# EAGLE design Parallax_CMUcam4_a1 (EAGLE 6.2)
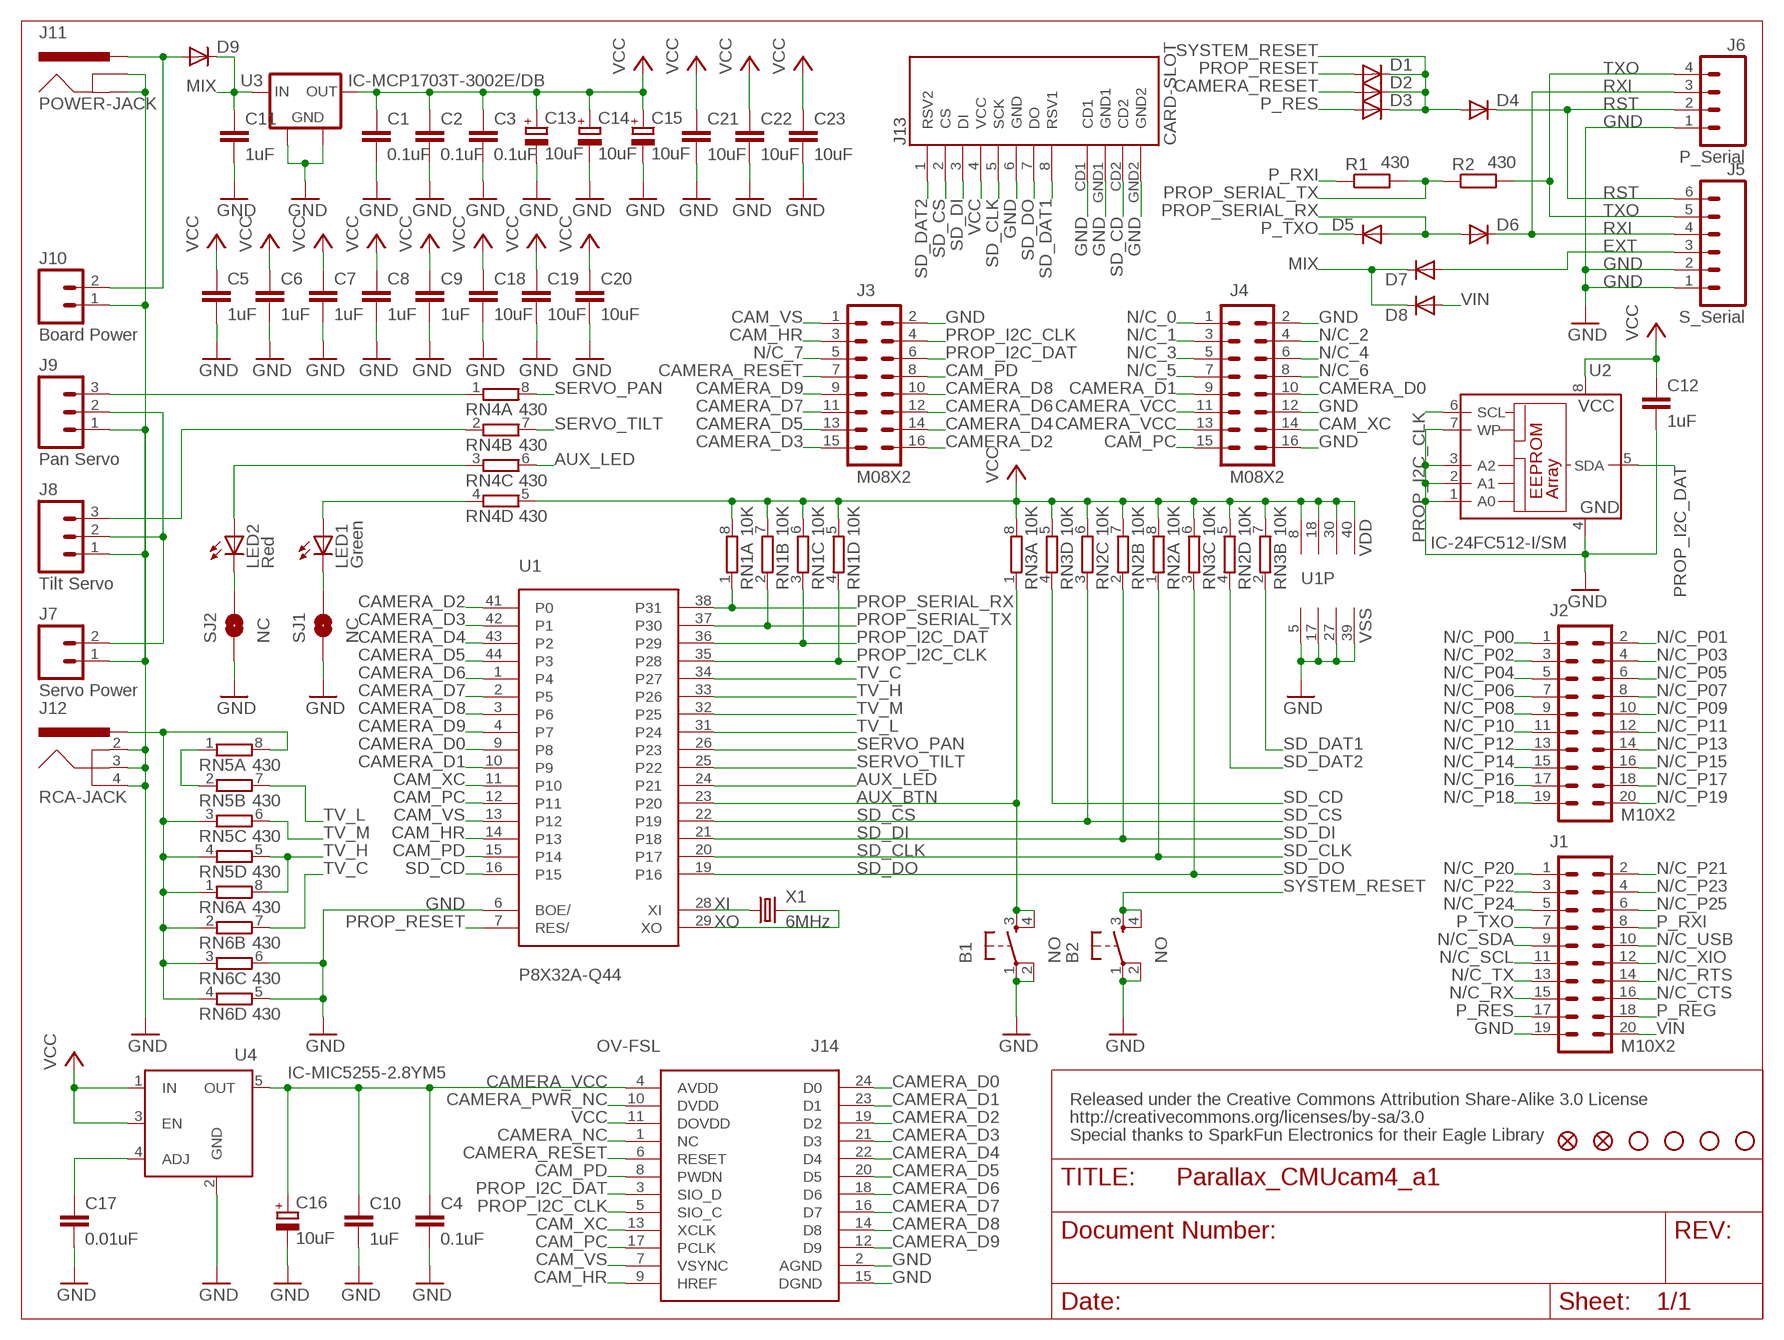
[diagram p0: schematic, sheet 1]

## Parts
B1  NO  PUSH-BUTTON  [PUSH-BUTTON]
B2  NO  PUSH-BUTTON  [PUSH-BUTTON]
C1  0.1uF  C-EUC0603K  [C0603K]
C2  0.1uF  C-EUC0603K  [C0603K]
C3  0.1uF  C-EUC0603K  [C0603K]
C4  0.1uF  C-EUC0603K  [C0603K]
C5  1uF  C-EUC0603K  [C0603K]
C6  1uF  C-EUC0603K  [C0603K]
C7  1uF  C-EUC0603K  [C0603K]
C8  1uF  C-EUC0603K  [C0603K]
C9  1uF  C-EUC0603K  [C0603K]
C10  1uF  C-EUC0603K  [C0603K]
C11  1uF  C-EUC0603K  [C0603K]
C12  1uF  C-EUC0603K  [C0603K]
C13  10uF  CPOL-EUA/3216-18R  [A/3216-18R]
C14  10uF  CPOL-EUA/3216-18R  [A/3216-18R]
C15  10uF  CPOL-EUA/3216-18R  [A/3216-18R]
C16  10uF  CPOL-EUA/3216-18R  [A/3216-18R]
C17  0.01uF  C-EUC0603K  [C0603K]
C18  10uF  C-EUC0603K  [C0603K]
C19  10uF  C-EUC0603K  [C0603K]
C20  10uF  C-EUC0603K  [C0603K]
C21  10uF  C-EUC0603K  [C0603K]
C22  10uF  C-EUC0603K  [C0603K]
C23  10uF  C-EUC0603K  [C0603K]
D1  DIODE-SOD523  [SOD523]
D2  DIODE-SOD523  [SOD523]
D3  DIODE-SOD523  [SOD523]
D4  DIODE-SOD523  [SOD523]
D5  DIODE-SOD523  [SOD523]
D6  DIODE-SOD523  [SOD523]
D7  DIODE-SOD323-R  [SOD323]
D8  DIODE-SOD323-R  [SOD323]
D9  DIODE-SOD323-R  [SOD323]
FID1  FIDUCIAL1X2  [FIDUCIAL-1X2]
FID2  FIDUCIAL1X2  [FIDUCIAL-1X2]
J1  M10X2  [2X10]
J2  M10X2  [2X10]
J3  M08X2  [2X8]
J4  M08X2  [2X8]
J5  S_Serial  M06SIP  [1X06]
J6  P_Serial  M04PTH  [1X04]
J7  Servo Power  M02PTH  [1X02]
J8  Tilt Servo  M03PTH  [1X03]
J9  Pan Servo  M03PTH  [1X03]
J10  Board Power  M02PTH  [1X02]
J11  POWER-JACK  [POWER-JACK]
J12  RCA-JACK  [RCA-JACK]
J13  CARD-SLOT  [CARD-SLOT]
J14  OV-FSL  [OV-FSL]
LED1  Green  LEDCHIP-LED0603  [CHIP-LED0603]
LED2  Red  LEDCHIP-LED0603  [CHIP-LED0603]
R1  430  R-EU_R0603  [R0603]
R2  430  R-EU_R0603  [R0603]
RN1  10K  4R-N0603-ARV  [0603-ARV]
RN2  10K  4R-N0603-ARV  [0603-ARV]
RN3  10K  4R-N0603-ARV  [0603-ARV]
RN4  430  4R-N0603-ARV  [0603-ARV]
RN5  430  4R-N0603-ARV  [0603-ARV]
RN6  430  4R-N0603-ARV  [0603-ARV]
SJ1  NC  SOLDERJUMPERTRACE  [SJ_2S-TRACE]
SJ2  NC  SOLDERJUMPERTRACE  [SJ_2S-TRACE]
STD1  STAND-OFF  [STAND-OFF]
STD2  STAND-OFF  [STAND-OFF]
STD3  STAND-OFF  [STAND-OFF]
STD4  STAND-OFF  [STAND-OFF]
U1  P8X32A-Q44  [P8X32A-Q44]
U2  IC-24FC512-I/SM  [IC-SO-08M]
U3  IC-MCP1703T-3002E/DB  [IC-SOT-223]
U4  IC-MIC5255-2.8YM5  [IC-SOT-23-5]
X1  6MHz  CRYSTALHC49UP  [HC49UP]

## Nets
AUX_BTN: B1.3 B1.4 RN3.1 U1.23(P20)
AUX_LED: RN4.6 U1.24(P21)
BYP: C17.1 U4.4(ADJ)
CAM_HR: J3.3 J14.9(HREF) U1.14(P13)
CAM_PC: J4.15 J14.17(PCLK) U1.12(P11)
CAM_PD: J3.8 J14.8(PWDN) U1.15(P14)
CAM_VS: J3.1 J14.7(VSYNC) U1.13(P12)
CAM_XC: J4.14 J14.13(XCLK) U1.11(P10)
CAMERA_D0: J4.10 J14.24(D0) U1.9(P8)
CAMERA_D1: J4.9 J14.23(D1) U1.10(P9)
CAMERA_D2: J3.16 J14.19(D2) U1.41(P0)
CAMERA_D3: J3.15 J14.21(D3) U1.42(P1)
CAMERA_D4: J3.14 J14.22(D4) U1.43(P2)
CAMERA_D5: J3.13 J14.20(D5) U1.44(P3)
CAMERA_D6: J3.12 J14.18(D6) U1.1(P4)
CAMERA_D7: J3.11 J14.16(D7) U1.2(P5)
CAMERA_D8: J3.10 J14.14(D8) U1.3(P6)
CAMERA_D9: J3.9 J14.12(D9) U1.4(P7)
CAMERA_NC: J14.1(NC)
CAMERA_PWR_NC: J14.10(DVDD)
CAMERA_RESET: D2.A J3.7 J14.6(RESET)
CAMERA_VCC: C4.1 C10.1 C16.+ J4.11 J4.13 J14.4(AVDD) U4.5(OUT)
EXT: D7.A J5.3
GND [vcc]: B1.1 B1.2 B2.1 B2.2 C1.2 C2.2 C3.2 C4.2 C5.2 C6.2 C7.2 C8.2 C9.2 C10.2 C11.2 C12.2 C13.- C14.- C15.- C16.- C17.2 C18.2 C19.2 C20.2 C21.2 C22.2 C23.2 J1.19 J3.2 J4.2 J4.12 J4.16 J5.1 J5.2 J6.1 J7.1 J8.1 J9.1 J10.1 J11.GND J11.GNDBREAK J12.2 J12.3 J12.4 J13.6(GND) J13.CD1 J13.GND1 J13.GND2 J14.2(AGND) J14.15(DGND) RN6.5 RN6.6 SJ1.1 SJ2.1 U1.5(VSS) U1.6(BOE/) U1.17(VSS) U1.27(VSS) U1.39(VSS) U2.1(A0) U2.2(A1) U2.3(A2) U2.4(GND) U2.7(WP) U3.2(GND) U3.4(FGND) U4.2(GND)
GREEN_BRIDGE: LED1.C SJ1.2
GREEN_CTRL: LED1.A RN4.4
MIX: C11.1 D7.C D8.C D9.C U3.1(IN)
N/C_0: J4.1
N/C_1: J4.3
N/C_2: J4.4
N/C_3: J4.5
N/C_4: J4.6
N/C_5: J4.7
N/C_6: J4.8
N/C_7: J3.5
N/C_CTS: J1.16
N/C_P00: J2.1
N/C_P01: J2.2
N/C_P02: J2.3
N/C_P03: J2.4
N/C_P04: J2.5
N/C_P05: J2.6
N/C_P06: J2.7
N/C_P07: J2.8
N/C_P08: J2.9
N/C_P09: J2.10
N/C_P10: J2.11
N/C_P11: J2.12
N/C_P12: J2.13
N/C_P13: J2.14
N/C_P14: J2.15
N/C_P15: J2.16
N/C_P16: J2.17
N/C_P17: J2.18
N/C_P18: J2.19
N/C_P19: J2.20
N/C_P20: J1.1
N/C_P21: J1.2
N/C_P22: J1.3
N/C_P23: J1.4
N/C_P24: J1.5
N/C_P25: J1.6
N/C_RTS: J1.14
N/C_RX: J1.15
N/C_SCL: J1.11
N/C_SDA: J1.9
N/C_TX: J1.13
N/C_USB: J1.10
N/C_XIO: J1.12
P_REG: J1.18
P_RES: D3.A J1.17
P_RXI: J1.8 R1.1
P_TXO: D5.C J1.7
PROP_I2C_CLK: J3.4 J14.5(SIO_C) RN1.4 U1.35(P28) U2.6(SCL)
PROP_I2C_DAT: J3.6 J14.3(SIO_D) RN1.3 U1.36(P29) U2.5(SDA)
PROP_RESET: D1.A U1.7(RES/)
PROP_SERIAL_RX: D5.A D6.A RN1.1 U1.38(P31)
PROP_SERIAL_TX: R1.2 R2.1 RN1.2 U1.37(P30)
RED_BRIDGE: LED2.C SJ2.2
RED_CTRL: LED2.A RN4.3
RST: D4.C J5.6 J6.2
RXI: D6.C J5.4 J6.3
SD_CD: J13.CD2 RN3.4 U1.16(P15)
SD_CLK: J13.5(SCK) RN2.1 U1.20(P17)
SD_CS: J13.2(CS) RN2.3 U1.22(P19)
SD_DAT1: J13.8(RSV1) RN3.2
SD_DAT2: J13.1(RSV2) RN2.4
SD_DI: J13.3(DI) RN2.2 U1.21(P18)
SD_DO: J13.7(DO) RN3.3 U1.19(P16)
SERVO_PAN: RN4.8 U1.26(P23)
SERVO_PAN_IO: J9.3 RN4.1
SERVO_PWR: J7.2 J8.2 J9.2
SERVO_TILT: RN4.7 U1.25(P22)
SERVO_TILT_IO: J8.3 RN4.2
SYSTEM_RESET: B2.3 B2.4 D1.C D2.C D3.C D4.A
SYSTEM_VIN: D9.A J10.2 J11.PWR
TV: J12.1 RN5.3 RN5.4 RN5.8 RN6.1 RN6.2 RN6.3 RN6.4
TV_C: RN6.7 U1.34(P27)
TV_H: RN5.5 RN6.8 U1.33(P26)
TV_L: RN5.7 U1.31(P24)
TV_M: RN5.6 U1.32(P25)
TV_R: RN5.1 RN5.2
TXO: J5.5 J6.4 R2.2
VCC: C1.1 C2.1 C3.1 C5.1 C6.1 C7.1 C8.1 C9.1 C12.1 C13.+ C14.+ C15.+ C18.1 C19.1 C20.1 C21.1 C22.1 C23.1 J13.4(VCC) J14.11(DOVDD) RN1.5 RN1.6 RN1.7 RN1.8 RN2.5 RN2.6 RN2.7 RN2.8 RN3.5 RN3.6 RN3.7 RN3.8 RN4.5 U1.8(VDD) U1.18(VDD) U1.30(VDD) U1.40(VDD) U2.8(VCC) U3.3(OUT) U4.1(IN) U4.3(EN)
VIN: D8.A J1.20
XI: U1.28(XI) X1.1
XO: U1.29(XO) X1.2

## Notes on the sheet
- Released under the Creative Commons Attribution Share-Alike 3.0 License
- http://creativecommons.org/licenses/by-sa/3.0
- Special thanks to SparkFun Electronics for their Eagle Library

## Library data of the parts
B1 B2 = custom-jacks:PUSH-BUTTON
C1-C12 C17-C23 = resistor:C-EU: CAPACITOR, European symbol
C13-C16 = resistor:CPOL-EU: POLARIZED CAPACITOR, European symbol
D1-D9 = diode:DIODE-: DIODE
FID1 FID2 = SparkFun:FIDUCIAL: Fiducial Alignment Points
J1 J2 = SparkFun-Connectors:M10X2: This was SPECIALLY designed to be used with our Graphic LCD Backpack. Be sure you want to use this! It is not only staggered on each line of header holes, but IT IS ALSO offset of the center point of the top and bottom lines by 5 mil. This causes the headers to lock into place on the "standard"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
J3 J4 = SparkFun-Connectors:M08X2: .1" headers, two rows of 8 each
J5 = SparkFun:M06: Header 6 Standard 6-pin 0.1" header. Use with straight break away headers (SKU : PRT-00116), right angle break away headers (PRT-00553), swiss pins (PRT-00743), machine pins (PRT-00117), and female headers (PRT-00115). Molex polarized connector foot print use with SKU : PRT-08094 with associated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
J6 = SparkFun:M04: Header 4 Standard 4-pin 0.1" header. Use with straight break away headers (SKU : PRT-00116), right angle break away headers (PRT-00553), swiss pins (PRT-00743), machine pins (PRT-00117), and female headers (PRT-00115). Molex polarized connector foot print use with SKU : PRT-08231 with associated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
J7 J10 = SparkFun:M02: Header 2
J8 J9 = SparkFun:M03: Header 3 Standard 3-pin 0.1" header. Use with straight break away headers (SKU : PRT-00116), right angle break away headers (PRT-00553), swiss pins (PRT-00743), machine pins (PRT-00117), and female headers (PRT-00115). Molex polarized connector foot print use with SKU : PRT-08232 with associated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
J11 = custom-jacks:POWER-JACK
J12 = custom-jacks:RCA-JACK
J13 = custom-jacks:CARD-SLOT
J14 = ovt-breakout:OV-FSL
LED1 LED2 = led:LED: LED
R1 R2 = resistor:R-EU_: RESISTOR, European symbol
RN1-RN6 = resistor-dil:4R-N: Array Chip Resistor Source: RS Component / Phycomp; OC_FARNELL: unknown; OC_NEWARK: unknown
SJ1 SJ2 = SparkFun:SOLDERJUMPER: Solder Jumper
STD1-STD4 = SparkFun:STAND-OFF: Stand Off
U1 = parallax-propeller:P8X32A-Q44
U2 = custom-jacks:IC-24FC512-I/SM
U3 = custom-jacks:IC-MCP1703T-3002E/DB
U4 = custom-jacks:IC-MIC5255-2.8YM5
X1 = crystal:CRYSTAL: CRYSTAL; OC_FARNELL: unknown; OC_NEWARK: unknown

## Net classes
0 default: width 0.203 mm
1 vcc: width 0.254 mm

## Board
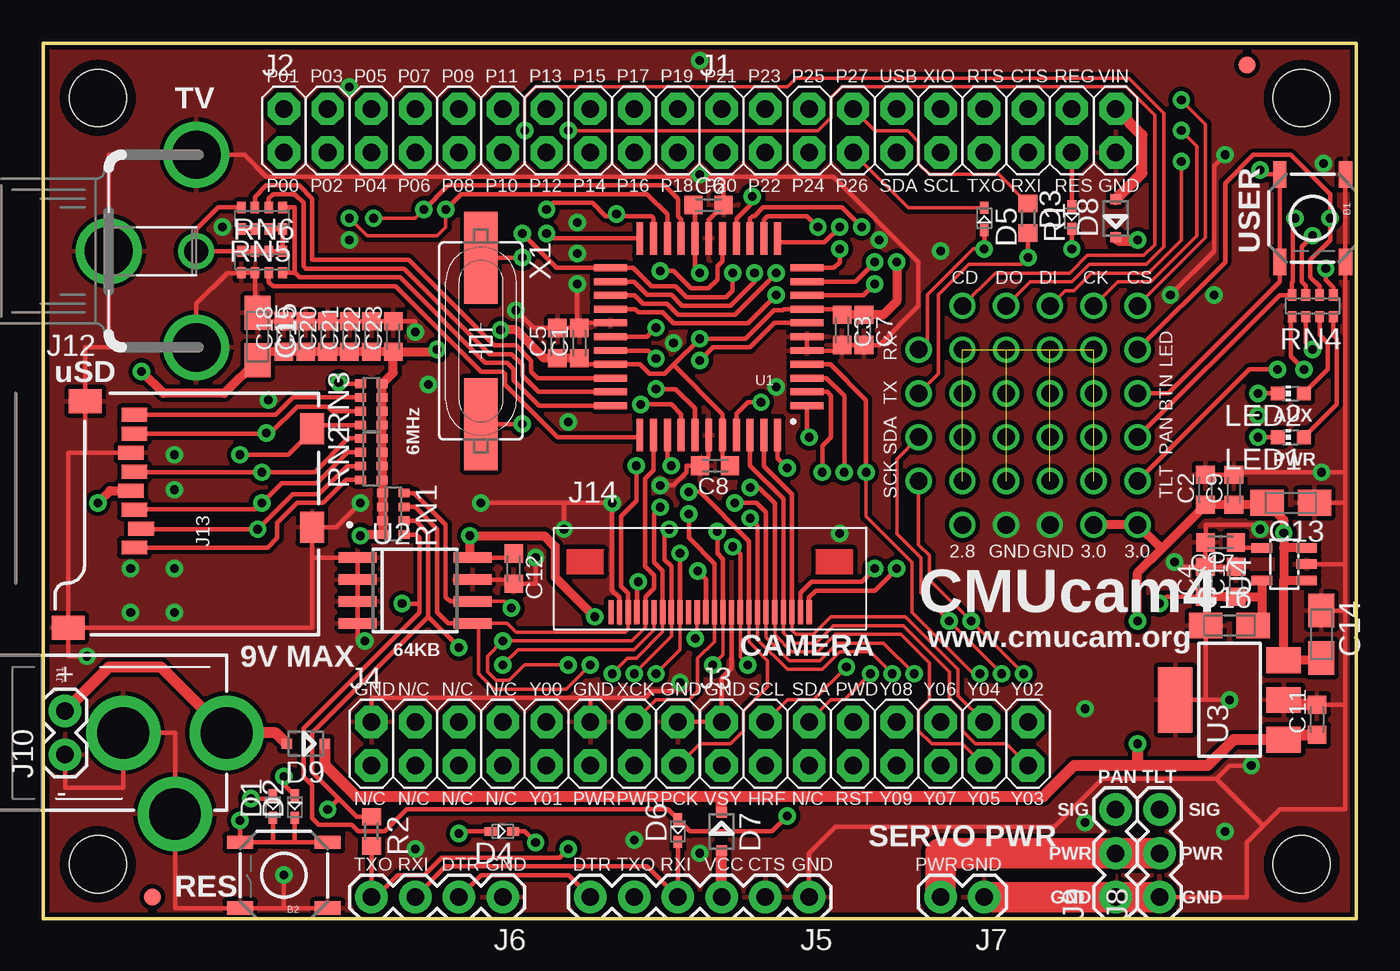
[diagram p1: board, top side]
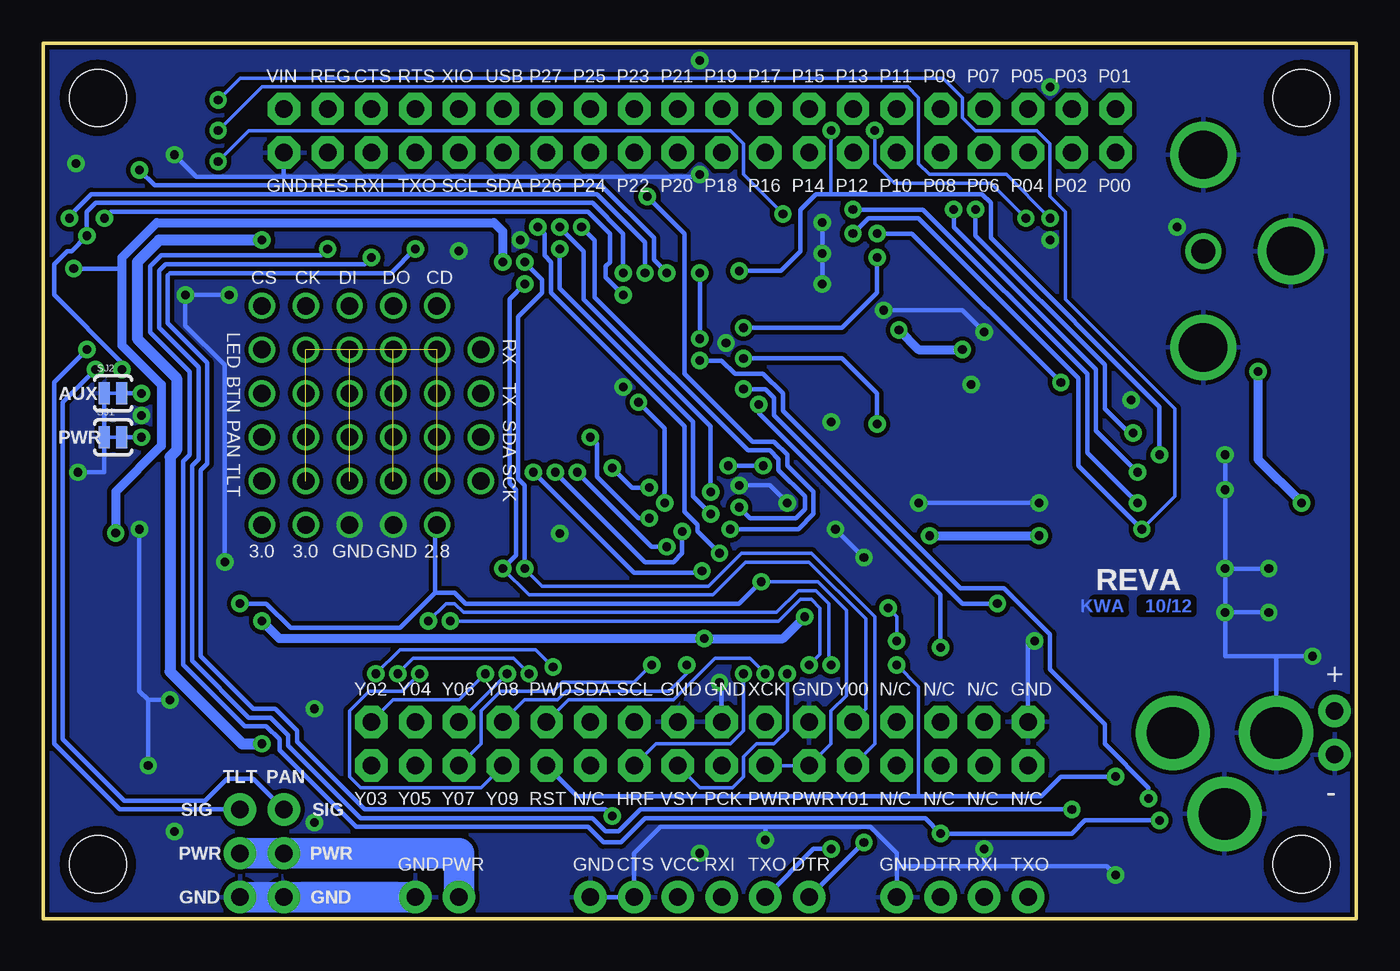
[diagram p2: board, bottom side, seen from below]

Size 76.2 x 50.8 mm. Coordinates in mm from the lower left corner, seen from the top.
Outline: 0,50.8 0,0 76.2,0 76.2,50.8 0,50.8
Copper layers (1*16): Top 0.035mm / dielectric 1.5mm / Bottom 0.035mm
Design rules: minimum track width 8mil, minimum drill 20mil, track to track 8mil, track to pad 8mil, pad to pad 8mil, via to via 8mil, smd to smd 8mil, copper to edge 10mil, drill to drill 8mil, minimum pad ring 12mil, minimum via ring 10mil, stop-mask expansion 4mil, vias tented up to drill 25mil, thermal gap 10mil
tRestrict: area 2,10.5 to 2.3,11; area 34.2,34.3 to 34.5,34.8; area 55,2.4 to 62,2.7; area 72.5,11.3 to 73.3,11.8; area 68.6,17.5 to 69.1,17.9; area 72.3,23.5 to 72.5,23.6; area 13,33.7 to 13.1,33.9; area 38.5,40.9 to 38.7,41
bRestrict: area 2,10.5 to 2.3,11; area 55,2.4 to 62,2.7

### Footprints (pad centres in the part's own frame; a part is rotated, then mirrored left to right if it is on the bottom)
PUSH-BUTTON = smd 1.524 x 0.762: 1 -2.54,1.905; 2 2.54,1.905; 3 -2.54,-1.905; 4 2.54,-1.905
C0603K = smd 1.05 x 1.08: 1 -0.875,0; 2 0.875,0
A/3216-18R = smd 1.95 x 1.5: + 1.375,0; - -1.375,0
SOD523 = smd 0.7 x 0.5: A 0.7,0; C -0.6,0
SOD323 = smd 0.6 x 0.6: A 1.1,0; C -1.1,0
FIDUCIAL-1X2 = smd 1 x 1: 1 0,0
2X10 = drill 1.016 pad 1.88 octagon: 1 -11.43,-1.27; 2 -11.43,1.27; 3 -8.89,-1.27; 4 -8.89,1.27; 5 -6.35,-1.27; 6 -6.35,1.27; 7 -3.81,-1.27; 8 -3.81,1.27; 9 -1.27,-1.27; 10 -1.27,1.27; 11 1.27,-1.27; 12 1.27,1.27; 13 3.81,-1.27; 14 3.81,1.27; 15 6.35,-1.27; 16 6.35,1.27; 17 8.89,-1.27; 18 8.89,1.27; 19 11.43,-1.27; 20 11.43,1.27
2X8 = drill 1.016 pad 1.88 octagon: 1 0,0; 2 0,2.54; 3 2.54,0; 4 2.54,2.54; 5 5.08,0; 6 5.08,2.54; 7 7.62,0; 8 7.62,2.54; 9 10.16,0; 10 10.16,2.54; 11 12.7,0; 12 12.7,2.54; 13 15.24,0; 14 15.24,2.54; 15 17.78,0; 16 17.78,2.54
1X06 = drill 1.016 pad 1.88: 1 0,0; 2 2.54,0; 3 5.08,0; 4 7.62,0; 5 10.16,0; 6 12.7,0
1X04 = drill 1.016 pad 1.88: 1 0,0; 2 2.54,0; 3 5.08,0; 4 7.62,0
1X02 = drill 1.016 pad 1.88: 1 0,0; 2 2.54,0
1X03 = drill 1.016 pad 1.88: 1 0,0; 2 2.54,0; 3 5.08,0
POWER-JACK = drill 2.997 pad 4.318: GND 0,7.7; GNDBREAK 4.7,10.7; PWR 0,13.7
RCA-JACK = drill 1.4: 1 0,0 | drill 2.8: 2 -5.588,0; 3 0,5.08; 4 5.588,0
CARD-SLOT = smd 0.8 x 1.5: 1 -8.94,10.7; 2 -7.84,10.3; 3 -6.74,10.7; 4 -5.64,10.9; 5 -4.54,10.7; 6 -3.44,10.9; 7 -2.34,10.7; 8 -1.24,10.7 | smd 1.8 x 1.4: CD1 -7.75,0.4; CD2 -2.05,0.4 | smd 1.4 x 1.9: GND1 -13.6,14.55; GND2 -0.45,13.55
OV-FSL = smd 0.3 x 1.4: 1 -5.15,-2.54; 2 -4.65,-2.54; 3 -4.15,-2.54; 4 -3.65,-2.54; 5 -3.15,-2.54; 6 -2.65,-2.54; 7 -2.15,-2.54; 8 -1.65,-2.54; 9 -1.15,-2.54; 10 -0.65,-2.54; 11 -0.15,-2.54; 12 0.35,-2.54; 13 0.85,-2.54; 14 1.35,-2.54; 15 1.85,-2.54; 16 2.35,-2.54; 17 2.85,-2.54; 18 3.35,-2.54; 19 3.85,-2.54; 20 4.35,-2.54; 21 4.85,-2.54; 22 5.35,-2.54; 23 5.85,-2.54; 24 6.35,-2.54
CHIP-LED0603 = smd 0.8 x 0.8: A 0,-0.75; C 0,0.75
R0603 = smd 1 x 1.1: 1 -0.85,0; 2 0.85,0
0603-ARV = smd 0.5 x 0.65: 1 -1.2,-0.625; 2 -0.4,-0.625; 3 0.4,-0.625; 4 1.2,-0.625; 5 1.2,0.625; 6 0.4,0.625; 7 -0.4,0.625; 8 -1.2,0.625
SJ_2S-TRACE = smd 0.635 x 1.27: 1 -0.508,0; 2 0.508,0
STAND-OFF = hole 3.302: 0,0
P8X32A-Q44 = smd 1.9 x 0.4: 1 -5.713,4.013; 2 -5.713,3.212; 3 -5.713,2.413; 4 -5.713,1.613; 5 -5.713,0.812; 6 -5.713,0.013; 7 -5.713,-0.787; 8 -5.713,-1.587; 9 -5.713,-2.388; 10 -5.713,-3.188; 11 -5.713,-3.987; 23 5.688,-3.987; 24 5.688,-3.188; 25 5.688,-2.388; 26 5.688,-1.587; 27 5.688,-0.787; 28 5.688,0.013; 29 5.688,0.812; 30 5.688,1.613; 31 5.688,2.413; 32 5.688,3.212; 33 5.688,4.013 | smd 0.4 x 1.9: 12 -4.013,-5.688; 13 -3.212,-5.688; 14 -2.413,-5.688; 15 -1.613,-5.688; 16 -0.812,-5.688; 17 -0.013,-5.688; 18 0.787,-5.688; 19 1.587,-5.688; 20 2.388,-5.688; 21 3.188,-5.688; 22 3.987,-5.688; 34 3.987,5.713; 35 3.188,5.713; 36 2.388,5.713; 37 1.587,5.713; 38 0.787,5.713; 39 -0.013,5.713; 40 -0.812,5.713; 41 -1.613,5.713; 42 -2.413,5.713; 43 -3.212,5.713; 44 -4.013,5.713
IC-SO-08M = smd 0.6 x 2.2: 1 -1.905,-3.33; 2 -0.635,-3.33; 3 0.635,-3.33; 4 1.905,-3.33; 5 1.905,3.33; 6 0.635,3.33; 7 -0.635,3.33; 8 -1.905,3.33
IC-SOT-223 = smd 1.5 x 2: 1 -2.3,-3.15; 2 0,-3.15; 3 2.3,-3.15 | smd 3.8 x 2: 4 0,3.15
IC-SOT-23-5 = smd 0.55 x 1.2: 1 -0.95,-1.3; 2 0,-1.3; 3 0.95,-1.3; 4 0.95,1.3; 5 -0.95,1.3
HC49UP = smd 5.334 x 1.93: 1 -4.826,0; 2 4.826,0

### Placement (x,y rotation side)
B1  73.66,40.64 270 top
B2  13.97,2.54 180 top
C1  31.11,33.4 90 top
C2  67.44,24.89 90 top
C3  46.35,34.16 270 top
C4  67.44,19.56 90 top
C5  29.84,33.4 90 top
C6  38.61,41.4 0 top
C7  47.62,34.16 270 top
C8  38.99,26.29 180 top
C9  69.09,24.89 90 top
C10  69.22,19.56 90 top
C11  73.91,11.56 90 top
C12  27.3,20.32 270 top
C13  72.39,24.13 180 top
C14  74.17,16.51 270 top
C15  12.45,33.78 270 top
C16  68.83,17.02 0 top
C17  68.33,21.84 180 top
C18  13.97,33.78 90 top
C19  15.24,33.78 90 top
C20  16.51,33.78 90 top
C21  17.78,33.78 90 top
C22  19.05,33.78 90 top
C23  20.32,33.78 90 top
D1  13.34,6.48 90 top
D2  14.61,6.48 90 top
D3  59.69,40.64 90 top
D4  26.67,5.08 180 top
D5  54.61,40.64 270 top
D6  36.83,5.08 90 top
D7  39.37,5.08 270 top
D8  62.23,40.64 90 top
D9  15.24,10.16 180 top
FID1  69.85,49.53 0 top
FID2  6.35,1.27 0 top
J1  50.8,45.72 0 top
J2  25.4,45.72 0 top
J3  39.37,8.89 0 top
J4  19.05,8.89 0 top
J5  44.45,1.27 180 top
J6  26.67,1.27 180 top
J7  54.61,1.27 180 top
J8  64.77,1.27 90 top
J9  62.23,1.27 90 top
J10  1.27,9.53 90 top
J11  -3.05,10.79 270 top
J12  8.89,38.73 90 top
J13  16,30.48 90 top
J14  38.1,20.32 0 top
LED1  72.39,27.94 90 top
LED2  72.39,30.48 90 top
R1  57.15,40.64 270 top
R2  19.05,5.08 270 top
RN1  20.32,23.5 90 top
RN2  19.05,26.67 270 top
RN3  19.05,29.84 270 top
RN4  73.66,35.56 0 top
RN5  12.7,40.64 0 top
RN6  12.7,38.1 180 top
SJ1  72.14,27.94 0 bottom
SJ2  72.14,30.48 0 bottom
STD1  3.17,47.62 0 top
STD2  73.03,3.17 0 top
STD3  73.03,47.62 0 top
STD4  3.17,3.17 0 top
U1  38.61,33.78 180 top
U2  21.59,19.05 270 top
U3  68.83,12.7 90 top
U4  72.01,20.57 90 top
X1  25.4,33.53 270 top

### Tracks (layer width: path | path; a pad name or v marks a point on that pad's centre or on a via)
AUX_BTN  (via drill 0.5, 1.02)
  Top 0.254: v17.14,31.11 17.21,31.05 RN3.1 | v40.01,37.47 40.01,36.45 39.62,36.07 37.34,36.07 36.7,36.7 35.31,36.7 34.24,37.77 U1.23 29.79,37.77 v27.81,39.75 | B1.3 B1.4 71.75,36.96 65.28,30.48 v63.5,30.48 | 71.75,43.05 B1.3 | v70.61,43.43 70.87,43.18 B1.3
  Bottom 0.254: v17.14,31.11 25.78,39.75 v27.81,39.75 | v40.01,37.47 40.77,38.23 40.77,39.5 43.81,42.55 69.72,42.55 v70.61,43.43
AUX_LED  (via drill 0.5, 1.02)
  Top 0.254: v41.27,37.47 41.27,36.96 39.88,35.56 37.08,35.56 36.45,36.2 35.05,36.2 34.28,36.97 U1.24 | RN4.6 74.06,36.68 73.53,37.21 73.53,38.23 74.68,39.37 v74.68,40.64 74.68,42.04 72.39,44.32 70.23,44.32 68.58,42.67 68.58,38.1 v63.5,33.02
  Bottom 0.254: v41.27,37.47 41.27,39.24 44.07,42.04 73.41,42.04 74.68,40.77 v74.68,40.64
BYP
  Top 0.254: U4.4 69.2,21.52 C17.1
CAM_HR  (via drill 0.5)
  Top 0.203: J14.9 36.95,15.61 v35.56,14.22
  Top 0.254: v47.5,40.13 46.35,41.27 41.78,41.27 41.27,40.77 41.15,40.77 41.02,40.64 U1.14 | J14.9 v36.95,21.2 v36.96,21.21
  Bottom 0.203: v35.56,14.22 35.56,10.92 36.32,10.16 40.64,10.16 J3.3
  Bottom 0.254: v36.96,21.21 38.23,22.48 38.23,22.86 38.99,23.62 38.99,28.57 46.74,36.32 46.74,38.1 47.12,38.48 47.12,39.75 v47.5,40.13
CAM_PC  (via drill 0.5)
  Top 0.203: J4.15 38.1,10.16 39.88,10.16 40.64,10.92 40.64,12.06 42.04,13.46 42.04,14.99 40.95,16.07 J14.17
  Top 0.254: J14.17 40.95,21.91 38.1,24.77 v37.47,24.77 | v46.23,40.13 45.34,39.24 42.62,39.24 U1.12
  Bottom 0.254: v37.47,24.77 37.47,28.57 44.83,35.94 44.83,38.73 v46.23,40.13
CAM_PD  (via drill 0.5)
  Top 0.203: J14.8 36.45,16.38 v34.29,14.22
  Top 0.254: J14.8 36.45,20.45 36.07,20.83 36.07,22.35 v36.32,22.61 | U1.15 40.22,40.6 41.15,41.53 v41.15,41.91
  Bottom 0.203: J3.8 45.72,12.7 39.62,12.7 37.21,15.11 35.18,15.11 v34.29,14.22
  Bottom 0.254: v36.32,22.61 32.38,22.61 31.5,23.5 31.5,24.77 33.02,26.29 33.02,26.92 33.78,27.69 35.05,27.69 38.99,31.62 38.99,39.75 v41.15,41.91
CAM_VS  (via drill 0.5)
  Top 0.203: J14.7 35.95,16.65 34.42,15.11 33.91,15.11 v33.02,14.22
  Top 0.254: v44.96,40.13 44.32,40.77 42.04,40.77 41.82,40.55 U1.13 | J14.7 35.95,20.18 35.43,20.7 35.43,23.5 v35.81,23.88
  Bottom 0.203: J3.1 38.1,7.62 36.2,7.62 35.56,8.26 35.56,9.4 34.8,10.16 33.78,10.16 33.02,10.92 v33.02,14.22
  Bottom 0.254: v44.96,40.13 44.2,39.37 44.2,36.07 35.31,27.18 34.04,27.18 33.53,26.67 33.53,26.04 32,24.51 32,23.75 32.51,23.24 35.18,23.24 v35.81,23.88
CAM_XC  (via drill 0.5)
  Top 0.203: J14.13 38.95,16.09 37.97,15.11 37.97,13.21 37.47,12.7 35.56,12.7 J4.14
  Top 0.254: J14.13 38.95,20.61 37.47,22.1 v37.47,23.5 | U1.11 45.9,37.77 46.23,38.1 v46.23,38.86
  Bottom 0.254: v46.23,38.86 46.23,36.58 38.48,28.83 38.48,24.51 v37.47,23.5
CAMERA_D0  (via drill 0.5)
  Top 0.254: J14.24 44.45,18.67 44.83,19.05 48.26,19.05 v49.53,20.32 | v48.26,36.83 47.6,36.17 U1.9
  Bottom 0.203: v49.53,20.32 48.01,18.8 37.34,18.8 35.43,20.7 31.75,20.7 28.45,17.4 28.45,12.19 J4.10
  Bottom 0.254: v49.53,20.32 48.77,21.08 48.77,24.89 49.15,25.27 49.15,35.94 v48.26,36.83
CAMERA_D1  (via drill 0.5)
  Top 0.254: J14.23 43.95,18.93 44.58,19.56 47.5,19.56 v48.26,20.32 | v48.26,38.1 47.13,36.97 U1.10
  Bottom 0.203: v48.26,20.32 47.24,19.3 37.59,19.3 35.69,21.21 31.62,21.21 27.94,17.53 27.94,10.16 J4.9
  Bottom 0.254: v48.26,20.32 48.26,25.15 48.64,25.53 48.64,34.92 47.24,36.32 47.24,37.08 v48.26,38.1
CAMERA_D2  (via drill 0.5)
  Top 0.203: J14.19 41.95,16.34 43.31,14.99 45.09,14.99 46.1,16 48.77,16 v50.55,14.22
  Top 0.254: J14.19 41.95,23.58 41.4,24.13 v40.13,24.13 | U1.41 40.22,29.3 40.89,29.97 v41.66,29.97
  Bottom 0.203: v50.55,14.22 52.07,12.7 55.88,12.7 J3.16
  Bottom 0.254: v41.66,29.97 40.13,28.45 v40.13,24.13
CAMERA_D3
  Top 0.203: J14.21 42.95,16.61 43.56,16 44.83,16 45.85,17.02 49.91,17.02 52.58,14.35 52.58,12.83 53.34,12.06 53.34,10.92 54.1,10.16 55.88,10.16 J3.15
  Top 0.254: U1.42 41.02,26.29 42.95,24.36 J14.21
CAMERA_D4
  Top 0.203: J14.22 43.45,16.75 43.69,16.51 44.7,16.51 45.72,17.53 50.04,17.53 53.09,14.48 53.09,12.95 J3.14
  Top 0.254: U1.43 41.82,26.25 43.45,24.62 J14.22
CAMERA_D5  (via drill 0.5)
  Top 0.203: J14.20 42.45,16.48 43.43,15.49 44.96,15.49 45.97,16.51 49.78,16.51 51.44,14.86 51.44,12.7 50.8,12.06 50.8,10.92 51.56,10.16 53.34,10.16 J3.13
  Top 0.254: J14.20 42.45,24.1 41.53,25.02 v41.02,25.02 | U1.44 42.62,26.72 v43.18,26.16
  Bottom 0.254: v41.02,25.02 42.04,25.02 v43.18,26.16
CAMERA_D6  (via drill 0.5)
  Top 0.203: J14.18 41.45,16.21 43.18,14.48 45.21,14.48 46.23,15.49 48.01,15.49 v49.28,14.22
  Top 0.254: J14.18 41.45,22.81 v41.02,23.24 | U1.1 44.32,28.07 v44.45,27.94
  Bottom 0.203: v49.28,14.22 J3.12
  Bottom 0.254: v41.02,23.24 41.66,23.24 44.07,25.65 44.07,27.56 v44.45,27.94
CAMERA_D7  (via drill 0.5)
  Top 0.203: J14.16 40.45,15.18 v40.89,14.73
  Top 0.254: J14.16 40.45,21.14 v40.01,21.59 | v45.21,25.91 45.21,27.43 45.72,27.94 45.72,30.35 45.5,30.57 U1.2
  Bottom 0.203: J3.11 50.8,10.16 50.8,12.06 49.66,13.21 46.61,13.21 46.1,13.72 41.91,13.72 v40.89,14.73
  Bottom 0.254: v40.01,21.59 40.89,21.59 v45.21,25.91
CAMERA_D8  (via drill 0.5)
  Top 0.203: J14.14 39.45,15.32 v38.86,14.73
  Top 0.254: J14.14 39.45,20.88 39.12,21.21 v39.12,22.48 | U1.3 45.47,31.37 46.48,30.35 v46.48,25.91
  Bottom 0.203: J3.10 48.26,12.7 46.35,12.7 45.85,13.21 39.88,13.21 38.86,14.22 v38.86,14.73
  Bottom 0.254: v39.12,22.48 39.12,21.21 39.62,20.7 41.27,20.7 v46.48,25.91
CAMERA_D9  (via drill 0.5)
  Top 0.203: v47.75,25.91 47.75,23.37 50.42,20.7 50.42,17.78 53.98,14.22 v54.36,14.22
  Top 0.254: J14.12 38.45,19.72 v37.97,20.19 | v47.75,25.91 47.75,30.1 45.68,32.17 U1.4
  Bottom 0.203: J3.9 50.8,7.62 57.78,7.62 58.42,8.26 58.42,12.06 57.28,13.21 55.37,13.21 v54.36,14.22
  Bottom 0.254: v37.97,20.19 38.1,20.07 41.91,20.07 v47.75,25.91
CAMERA_RESET  (via drill 0.5)
  Top 0.203: J14.6 35.45,16.78 34.29,15.62 27.56,15.62 v26.67,14.73
  Top 0.254: D2.A 13.97,7.81 v13.97,8.26
  Bottom 0.203: v26.67,14.73 25.4,13.46 25.4,7.11
  Bottom 0.254: v13.97,8.26 17.14,8.26 18.29,7.11 25.4,7.11 45.21,7.11 J3.7
CAMERA_VCC  (via drill 0.5, 1.02)
  Top 0.254: J14.4 34.45,19.46 v34.54,19.56 | 68.58,18.68 65.17,18.68 v64.77,18.29
  Top 0.508: U4.5 70.71,18.68 | C16.+ 70.71,17.02 70.71,18.68 | C4.1 68.58,18.68 C10.1 70.71,18.68
  Bottom 0.203: v34.54,19.56 31.24,19.56 29.59,17.91 29.59,12.95 30.48,12.06 30.48,10.16 J4.11 J4.13
  Bottom 0.254: v34.54,19.56 35.81,18.29 51.69,18.29 52.32,18.92 53.47,18.92 | 53.47,18.92 55.5,16.89 61.85,16.89 63.25,18.29 v64.77,18.29 | v53.34,22.86 53.47,22.73 53.47,18.92
EXT
  Top 0.635: J5.3 D7.A
GND  (via drill 0.5, 0.5 pad 0.2, 0.5 pad 0.25, 1.02)
  Top 0.254: B2.2 B2.1 | B2.2 13.97,0.64 v13.97,2.54 | B2.2 7.65,0.64 J11.GNDBREAK 7.65,10.79 J11.GND 4.65,7.62 1.27,7.62 J10.1 | J13.GND1 1.45,15.24 v2.54,15.24 | U2.7 27.3,19.68 C12.2 | 15.6,20.95 U2.1 U2.2 U2.3 U2.4 18.26,16.13 v18.67,16.13 | J13.GND1 15.6,16.88 15.6,20.95 | 2.45,27.04 J13.GND2 2.45,33.15 3.81,33.15 | 2.45,27.04 J13.6 | J13.GND1 1.45,27.04 2.45,27.04 | 3.81,33.15 J12.2 8.89,35.69 10.67,37.47 11.49,37.47 RN6.5 RN6.6 12.3,35.16 C15.- 12.45,34.66 C18.2 C19.2 C20.2 C21.2 C22.2 C23.2 20.33,34.67 21.59,34.67 v21.59,34.04 | 3.81,33.15 J12.3 3.81,44.32 J12.4 11.68,44.32 12.95,43.05 38.1,43.05 | U1.17 38.62,40.54 C6.2 39.48,43.04 39.5,43.05 | U1.27 31.11,34.57 C1.2 | C1.2 C5.2 28.45,34.29 v27.43,35.31 | 75.56,25.91 B1.2 B1.1 | 75.56,25.91 75.56,24.13 | 75.56,24.13 75.56,20.57 | 75.56,20.57 75.56,17.89 | 75.56,17.89 75.56,12.43 | 75.56,12.43 75.56,6.35 71.75,6.35 70.8,5.4 | J8.1 69.85,1.27 69.85,4.45 70.8,5.4 | J5.1 44.45,3.81 45.97,5.33 58.67,5.33 61.47,8.13 68.07,8.13 | 75.56,25.91 v74.17,25.91 69.09,25.91 C9.2 C2.2 | C14.- 75.56,17.89 | C11.2 75.56,12.43 | U3.4 v68.83,12.7 | v70.1,8.89 68.83,8.89 68.07,8.13 | C7.2 C3.2 46.35,32.97 U1.5 U1.6 | U3.4 65.68,13.87 | 65.53,12.7 U3.4 | U4.2 75.56,20.57 | C13.- 75.56,24.13 | C16.- 67.46,12.7 U3.4 | C10.2 C4.2 | v70.61,22.61 70.36,22.86 67.45,22.86 C17.2 67.44,21.83 C4.2 | 68.07,8.13 70.8,5.4 | 38.1,43.05 39.5,43.05 | U1.39 38.62,26.8 C8.2 37.34,26.29 37.34,25.91 36.58,25.15 v35.81,25.15 | v18.41,24.13 17.02,22.73 J13.CD1 15.6,20.95 | v25.4,24.13 30.23,24.13 | 30.23,24.13 v33.02,24.13 33.02,19.05 33.45,18.62 J14.2 | 47.62,33.27 C7.2 | C12.2 27.42,19.45 | v30.23,22.61 30.23,24.13
  Top 0.254: v28.57,20.95 28.57,19.45 C12.2 | J14.15 39.95,14.55 39.37,13.97 J3.2 J4.16 | v36.96,13.72 36.45,13.21 35.31,13.21 34.92,12.83 31.75,12.83 | 31.75,12.83 19.05,12.83 J4.2 | J4.12 31.75,12.83 | v30.99,36.83 30.99,34.29 C1.2 | v38.1,43.18 38.1,43.05 | 39.5,43.05 45.85,43.05 50.8,38.1 50.8,35.56 48.51,33.27 47.64,33.27 C7.2 | v68.58,44.32 67.94,43.69 67.94,38.73 v65.41,36.2 | C4.2 65.93,20.43 v65.66,20.7
  Top 0.635: C11.2 71.98,12.43 U3.2
  Top 1.778: J7.1 J9.1 J8.1
  Bottom 0.254: J6.1 26.67,3.05 | 34.29,5.33 28.19,5.33 26.67,3.81 26.67,3.05 | 34.29,5.33 40.39,5.33 41.91,3.81 J5.2 J5.1 | v13.97,2.54 14.48,3.05 21.59,3.05 | 21.59,3.05 26.67,3.05 | v2.54,15.24 4.65,15.24 | 4.65,15.24 J11.GND | v34.29,4.57 34.29,5.33 | v21.59,4.06 21.59,3.05 | SJ1.1 SJ2.1 72.64,25.91 v74.17,25.91 | v68.83,12.7 70.1,12.7 | 70.1,12.7 v70.1,8.89 | v70.61,22.61 70.61,13.21 70.1,12.7 | v27.43,35.31 22.86,35.31 v21.59,34.04 | v18.41,24.13 v25.4,24.13 | v18.67,16.13 19.05,16.13 J4.2 | v28.57,20.95 v30.23,22.61 | J4.16 36.83,13.59 v36.96,13.72 | 4.65,15.24 7.62,15.24 v7.62,24.89 v7.62,26.92 | v30.99,40.39 v30.99,38.61 v30.99,36.83 | v5.08,20.32 v7.62,20.32 | v5.08,17.78 v7.62,17.78 | v35.81,25.15 34.04,25.15 v33.02,24.13 | v38.1,43.18 38.23,43.05 62.23,43.05 | J1.19 62.23,43.05 | 62.23,43.05 67.31,43.05 v68.58,44.32 | v65.41,36.2 v67.94,36.2 67.94,34.42 65.66,32.13 v65.66,20.7
  Bottom 1.778: 54.74,1.27 J8.1
  other vias: 46.23,22.35 22.35,30.99 38.1,3.81 60.45,5.59 68.58,5.08 48.51,39.37 60.45,12.19 70.48,29.21 17.78,48.26 42.55,30.86 30.48,28.83 52.07,38.73 13.08,30.1 10.41,40.13 36.58,33.4 17.78,39.37 38.1,49.78 58.42,22.86 55.88,22.86 74.3,43.81
  pour Top (isolate 0.254): 0,50.8 76.2,50.8 76.2,0 0,0
  pour Bottom (isolate 0.254): 0,50.8 76.2,50.8 76.2,0 0,0
GREEN_BRIDGE  (via drill 0.5)
  Top 0.254: LED1.C v70.48,27.94
  Bottom 0.254: SJ1.2 v70.48,27.94
GREEN_CTRL
  Top 0.254: RN4.4 74.86,33.85 75.06,33.66 75.06,29.86 LED1.A
HOLE  (via drill 1.02)  (15 unrouted)
  other vias: 53.34,33.02 55.88,33.02 58.42,33.02 60.96,33.02 60.96,30.48 58.42,30.48 55.88,30.48 53.34,30.48 53.34,27.94 55.88,27.94 58.42,27.94 60.96,27.94 53.34,25.4 55.88,25.4 58.42,25.4 60.96,25.4
MIX  (via drill 0.5)
  Top 0.635: D9.C 16.34,8.93 18.16,7.11 39.37,7.11 | 39.37,7.11 58.04,7.11 59.82,8.89 63.5,8.89 | D7.C 39.37,7.11 | 63.5,8.89 67.56,8.89 69.07,10.4 U3.1 71.98,10.68 C11.1 | D8.C 62.4,39.37 v63.5,39.37 | v63.5,10.16 63.5,8.89
  Bottom 0.635: v63.5,39.37 69.47,39.37 70.74,38.1 70.74,33.66 68.45,31.37 68.45,27.18 68.83,26.8 68.83,14.35 64.64,10.16 v63.5,10.16
P_RES
  Top 0.254: J1.17 D3.A
P_RXI
  Top 0.203: R1.1 55.46,43.18 51.44,43.18 50.8,43.81 50.8,45.09 50.16,45.72 48.26,45.72 J1.8
P_TXO
  Top 0.203: D5.C 50.2,41.24 J1.7
PROP_I2C_CLK  (via drill 0.5, 0.5 pad 0.2, 1.02)
  Top 0.203: J14.5 34.95,16.92 34.16,16.13 v26.67,16.13 25.78,15.24 25.78,14.35 26.29,13.84 27.05,13.84 27.94,14.73 v30.48,14.73 | U2.6 26.8,18.41 v27.18,18.03 | J3.4 43.18,12.7 44.7,12.7 v46.61,14.61 | v56.9,14.22 v53.85,17.27 51.44,19.68 51.44,21.08 50.8,21.72 v50.8,25.4
  Top 0.254: U2.6 23.62,18.41 23.37,18.67 23.37,22.86 21.53,24.7 RN1.4 | U1.35 35.42,26.02 34.92,25.53 34.92,20.45 35.43,19.94 35.43,19.18 34.95,18.69 J14.5
  Bottom 0.203: v26.67,16.13 26.67,17.53 v27.18,18.03 | v46.61,14.61 47.62,15.62 55.5,15.62 v56.9,14.22 | v53.85,17.27 52.83,18.29 52.32,18.29 51.82,17.78 33.66,17.78 32.38,19.05 31.37,19.05 30.61,18.29 30.61,14.86 v30.48,14.73
PROP_I2C_DAT  (via drill 0.5, 0.5 pad 0.2, 1.02)
  Top 0.203: J14.3 33.95,16.8 33.78,16.64 27.43,16.64 26.92,17.14 U2.5 25.27,17.14 25.27,14.22 26.16,13.34 30.35,13.34 v31.75,14.73 | J3.6 45.72,12.7 46.48,12.7 v48.01,14.22 | v55.63,14.22 v52.58,17.27 50.93,18.92 50.93,20.95 49.53,22.35 49.53,26.67 v50.8,27.94
  Top 0.254: U2.5 23.5,17.14 22.86,17.78 22.86,22.61 21.57,23.89 RN1.3 | v34.42,26.29 34.42,24.26 33.53,23.37 33.53,19.3 33.95,18.88 J14.3 | U1.36 36.22,26.52 v36.45,26.29
  Bottom 0.203: v48.01,14.22 48.9,15.11 54.74,15.11 v55.63,14.22 | v52.58,17.27 33.53,17.27 32.26,18.54 31.62,18.54 31.11,18.03 31.11,15.37 v31.75,14.73
  Bottom 0.254: v36.45,26.29 v34.42,26.29
PROP_RESET  (via drill 0.5)
  Top 0.254: D1.A 13.14,6.99 v12.06,6.99 | v38.1,32.38 38.86,33.15 41.02,33.15 42.44,34.57 U1.7
  Bottom 0.254: v12.06,6.99 12.06,7.62 14.61,10.16 14.61,11.3 17.78,14.48 17.78,16.51 20.45,19.18 22.99,19.18 33.27,29.46 33.27,30.48 34.42,31.62 36.07,31.62 36.83,32.38 v38.1,32.38
PROP_SERIAL_RX  (via drill 0.5, 1.02)
  Top 0.203: v50.8,33.02 51.31,33.53 51.31,36.2 53.98,38.86 v54.61,38.86
  Top 0.254: RN1.1 21.65,22.3 21.84,22.1 21.84,18.29 | 21.84,18.29 21.84,17.78 15.11,11.05 15.11,8.26 15.62,7.75 15.62,5.84 16,5.46 17.91,5.46 18.29,5.08 19.81,5.08 21.08,6.35 36.26,6.35 D6.A 37.53,5.08 42.29,5.08 v43.18,5.97 | v20.83,18.29 21.84,18.29 | v35.56,30.73 36.7,30.73 37.82,29.62 U1.38 | D5.A v54.61,38.86
  Bottom 0.254: v35.56,30.73 34.29,30.73 33.78,30.23 33.78,29.21 22.86,18.29 v20.83,18.29 | v54.61,38.86 56.01,37.47 68.83,37.47 68.96,37.34 68.96,34.54 66.67,32.26 66.67,26.42 67.06,26.04 67.06,15.24 64.01,12.19 62.74,12.19 61.47,10.92 61.47,10.29 57.53,6.35 43.56,6.35 v43.18,5.97
PROP_SERIAL_TX  (via drill 0.5, 1.02)
  Top 0.203: v50.8,30.48 51.94,31.62 51.94,36.2 53.72,37.97 56.77,37.97 v57.15,38.35
  Top 0.254: R2.1 18.2,5.93 17.14,6.99 | 17.14,6.99 15.62,8.51 15.62,10.79 22.35,17.53 | 22.35,17.53 22.35,22.35 21.61,23.09 RN1.2 | U1.37 37.02,29.27 36.45,29.84 v34.67,29.84 | v24.13,15.75 22.35,17.53 | R1.2 v57.15,38.35 | v16.51,6.35 17.14,6.99
  Bottom 0.254: v34.67,29.84 34.67,29.34 24.13,18.8 v24.13,15.75 | v57.15,38.35 57.53,37.97 69.09,37.97 69.47,37.59 69.47,34.29 67.18,32 67.18,26.67 67.56,26.29 67.56,14.99 64.26,11.68 62.99,11.68 61.98,10.67 61.98,10.03 57.78,5.84 44.32,5.84 43.56,5.08 42.8,5.08 41.53,6.35 v16.51,6.35
RED_BRIDGE  (via drill 0.5)
  Top 0.254: LED2.C v70.48,30.48
  Bottom 0.254: SJ2.2 v70.48,30.48
RED_CTRL
  Top 0.254: RN4.3 74.06,33.89 74.55,33.4 74.55,31.89 LED2.A
RST  (via drill 0.5)
  Top 0.254: J6.2 25.4,2.54 30.48,2.54 J5.6 | v28.57,4.45 27.94,5.08 D4.C
  Bottom 0.254: J5.6 v28.57,4.45
RXI
  Top 0.254: J6.3 23.37,3.05 35.05,3.05 J5.4 D6.C
SD_CD  (via drill 0.5, 1.02)
  Top 0.203: v53.34,35.56 55.24,37.47 59.56,37.47 60.58,38.48 63.88,38.48 64.52,39.12 64.52,46.61 62.87,48.26 46.35,48.26 45.72,47.62 45.72,46.48 44.96,45.72 v30.48,45.72
  Top 0.254: RN3.4 15.6,28.64 J13.CD2 15.6,28.3 14.22,26.92 v11.43,26.92 | U1.16 39.42,38.15 39.12,37.85 39.12,37.08 38.61,36.58 37.59,36.58 36.58,37.59 v35.81,37.59
  Bottom 0.203: v30.48,45.72 30.48,42.04
  Bottom 0.254: v11.43,26.92 11.43,29.72 21.21,39.5 21.21,41.53 21.72,42.04 30.48,42.04 31.37,42.04 32.26,41.15 32.26,38.73 33.4,37.59 v35.81,37.59
SD_CLK  (via drill 0.5, 1.02)
  Top 0.203: 34.29,42.04 33.02,42.04 | v60.96,35.56 62.36,36.96 64.26,36.96 66.93,39.62 66.93,44.83 v66.04,45.72 | v17.78,40.64 18.8,39.62 22.86,39.62 23.37,40.13 v23.37,41.15
  Top 0.254: RN2.1 17.71,27.87 15.75,25.91 v12.7,25.91 | v12.7,25.91 5.3,25.91 J13.5 5.33,25.91 v12.7,25.91 | U1.20 36.22,40.87 35.05,42.04 33.02,42.04 24.26,42.04 v23.37,41.15
  Bottom 0.203: v66.04,45.72 63.5,48.26 26.04,48.26 25.4,47.62 25.4,43.81 24.77,43.18 20.32,43.18 v17.78,40.64
  Bottom 0.254: v23.37,41.15 23.37,40.13 15.11,31.88 15.11,28.32 v12.7,25.91
SD_CS  (via drill 0.5, 1.02)
  Top 0.203: v63.5,35.56 67.44,39.5 67.44,46.1 v66.04,47.5
  Top 0.254: RN2.3 17.63,26.27 16,24.64 14.48,24.64 v12.45,22.61 5.7,22.61 J13.2 | U1.22 29.49,39.47 v29.21,39.75
  Bottom 0.203: v66.04,47.5 64.77,48.77 24,48.77 22.86,47.62 22.86,46.48 22.1,45.72 18.54,45.72 17.78,44.96 17.78,41.91 16.89,41.02 16.89,35.94 10.54,29.59 10.54,24.51 v12.45,22.61
  Bottom 0.254: v29.21,39.75 28.32,40.64 25.4,40.64 16.13,31.37 16.13,26.29 v12.45,22.61
SD_DAT1
  Top 0.254: RN3.2 14.5,30.25 13.49,29.24 J13.8
SD_DAT2
  Top 0.254: RN2.4 17.6,25.47 16.26,24.13 14.73,24.13 13.59,22.99 13.59,22.1 13.03,21.54 J13.1
SD_DI  (via drill 0.5, 1.02)
  Top 0.203: v58.42,35.56 59.31,36.45 59.82,36.45 60.83,37.47 64.14,37.47 66.04,39.37 v66.04,43.94 | v33.27,40.89 33.27,40.77
  Top 0.254: RN2.2 17.67,27.07 15.88,25.27 13.84,25.27 v12.7,24.13 12.32,23.75 J13.3 | U1.21 35.42,40.65 35.31,40.77 33.27,40.77 32.64,40.77 31.88,41.53 29.59,41.53 v29.21,41.15
  Bottom 0.203: v66.04,43.94 64.26,45.72 36.32,45.72 35.56,44.96 35.56,43.18 v33.27,40.89
  Bottom 0.254: v29.21,41.15 25.15,41.15 15.62,31.62 15.62,27.05 v12.7,24.13
SD_DO  (via drill 0.5, 1.02)
  Top 0.203: v55.88,35.56 57.28,36.96 59.69,36.96 60.71,37.97 64.01,37.97 65.02,38.99 65.02,46.74 62.99,48.77 43.69,48.77 43.18,48.26 28.57,48.26 27.94,47.62 v27.94,45.72 | v19.18,40.64 21.59,40.64 v22.1,41.15
  Top 0.254: RN3.3 16.78,29.45 16.51,29.72 14.73,29.72 13.21,28.19 v12.95,28.19 12.9,28.14 J13.7 | U1.19 37.02,40.58 36.83,40.77 36.83,41.78 36.07,42.55 23.5,42.55 v22.1,41.15
  Bottom 0.203: v27.94,45.72 27.94,43.81 26.8,42.67 21.21,42.67 v19.18,40.64
  Bottom 0.254: v22.1,41.15 22.1,39.62 14.61,32.13 14.61,29.59 13.21,28.19 v12.95,28.19
SERVO_PAN  (via drill 0.5, 1.02)
  Top 0.254: v42.55,36.2 40.89,34.54 36.58,34.54 35.94,35.18 34.54,35.18 34.35,35.37 U1.26 | v72.64,40.64 72.52,40.51 72.52,36.96 72.46,36.9 RN4.8 71.75,36.19 v63.5,27.94
  Bottom 0.254: v42.55,36.2 43.56,37.21 43.56,37.85 43.31,38.1 43.31,39.75 44.58,41.02 72.26,41.02 v72.64,40.64
SERVO_PAN_IO  (via drill 0.5)
  Top 0.254: RN4.1 72.39,34.87 72.39,32.64 v73.15,31.88
  Bottom 0.254: v73.15,31.88 75.06,29.97 75.06,10.41 71.5,6.86 66.8,6.86 65.53,8.13 64.01,8.13 J9.3
SERVO_PWR
  Top 1.778: J8.2 J9.2 52.07,3.81 J7.2
  Bottom 1.778: J7.2 52.07,3.81 J9.2 J8.2
SERVO_TILT  (via drill 0.5, 1.02)
  Top 0.254: v42.55,37.47 40.13,35.05 36.83,35.05 36.2,35.69 34.8,35.69 34.32,36.17 U1.25 | v73.66,39.62 73.03,38.99 73.03,36.96 73.26,36.72 RN4.7 | v63.5,25.4 69.98,31.88 v71.63,31.88
  Bottom 0.254: v42.55,37.47 42.55,39.75 44.32,41.53 73.15,41.53 73.66,41.02 v73.66,39.62 74.55,38.73 74.8,38.73 75.56,37.97 75.56,36.2 71.63,32.26 v71.63,31.88
SERVO_TILT_IO  (via drill 0.5)
  Top 0.254: RN4.2 73.26,33.42 v73.66,33.02
  Bottom 0.254: v73.66,33.02 75.56,31.11 75.56,10.16 71.75,6.35 J8.3
SYSTEM_RESET  (via drill 0.5)
  Top 0.254: 14.61,4.45 13.34,4.45 D1.C | 14.61,4.45 B2.3 B2.4 v11.43,5.71 | D2.C 14.61,4.45 | D4.A 24.26,5.08 v24.13,4.95 | D3.C v59.69,38.86
  Bottom 0.254: v11.43,5.71 15.75,5.71 16.51,4.95 v24.13,4.95 25.02,5.84 41.27,5.84 42.67,4.45 43.69,4.45 44.58,5.33 58.04,5.33 62.48,9.78 62.48,10.41 63.25,11.18 64.52,11.18 68.07,14.73 68.07,26.54 67.69,26.92 67.69,31.75 69.98,34.04 69.98,37.85 69.34,38.48 60.07,38.48 v59.69,38.86
SYSTEM_VIN
  Top 0.635: J10.2 3.81,14.61 6.84,14.61 J11.PWR 13.51,10.79 D9.A
TV
  Top 0.254: RN5.3 RN5.4 RN6.1 RN6.2 RN6.3 RN6.4 J12.1 8.89,40.01 10.15,41.27 RN5.8
TV_C
  Top 0.254: RN6.7 13.1,36.94 13.34,36.7 20.45,36.7 25.4,31.75 26.67,31.75 26.8,31.62 26.8,30.99 29.84,27.94 34.62,27.94 U1.34
TV_H
  Top 0.254: RN6.8 14.61,37.48 | RN5.5 14.61,41.27 14.61,37.48 | U1.33 28.78,29.77 27.3,31.24 27.3,31.88 26.92,32.26 25.65,32.26 20.7,37.21 14.88,37.21 14.62,37.48 14.61,37.48
TV_L
  Top 0.254: U1.31 28.7,31.37 28.32,31.75 28.32,32.38 27.43,33.27 26.16,33.27 21.21,38.23 15.62,38.23 15.62,41.78 14.86,42.55 12.95,42.55 12.3,41.89 RN5.7
TV_M
  Top 0.254: U1.32 28.74,30.57 27.81,31.5 27.81,32.13 27.18,32.77 25.91,32.77 20.95,37.72 15.24,37.72 15.11,37.85 15.11,41.53 14.61,42.04 13.34,42.04 13.1,41.8 RN5.6
TV_R
  Top 0.254: RN5.1 RN5.2
TXO  (via drill 0.5)
  Top 0.254: v30.48,4.06 29.97,3.56 23.11,3.56 22.1,2.54 20.57,2.54 19.3,1.27 J6.4 R2.2
  Bottom 0.254: J5.5 31.5,4.06 v30.48,4.06
VCC  (via drill 0.5, 0.5 pad 0.25, 1.02)
  Top 0.203: J14.11 37.95,16.36 v37.85,16.26
  Top 0.254: C12.1 27.3,20.95 U2.8 | C1.1 31.11,32.17 U1.30 34.63,32.17 35.18,31.62 36.07,31.62 36.58,32.13 | C6.1 37.82,41.4 U1.18 37.82,37.74 v38.1,37.47 | C3.1 46.35,35.37 U1.8 42.99,35.37 42.93,35.31 42.42,35.31 40.77,33.66 v38.1,33.66 36.58,32.13 | RN4.5 74.86,36.65 74.42,37.08 v74.42,37.72 | 36.58,32.13 39.42,29.29 U1.40 39.42,26.73 C8.1
  Top 0.508: 24.92,22.23 v24.77,22.23 | v18.41,22.23 18.48,22.3 RN1.8 RN1.7 RN1.6 RN1.5 19.7,25.47 RN2.5 RN2.6 RN2.7 RN2.8 RN3.5 RN3.6 RN3.7 RN3.8 20.32,31.69 C23.1 | C23.1 C22.1 C21.1 C20.1 C19.1 C18.1 12.45,32.91 C15.+ 10.52,30.48 6.99,30.48 v5.71,31.75 | v3.17,24.13 3.88,24.84 J13.4 | C1.1 C5.1 29.07,32.53 27.43,34.16 v26.54,34.16 | 71.98,19.62 U3.3 74.17,15 C14.+ | C3.1 C7.1 48.75,35.04 49.53,35.81 v49.53,38.1 | U4.1 71.98,19.62 | U4.3 71.98,21.52 | 71.98,21.52 71.98,19.62 | 71.98,21.52 v71.98,22.38 71.98,23.16 C13.+ 71.02,24.02 C9.1 C2.1 | C23.1 22.75,32.91 v22.86,33.02 | v24.77,22.23 29.08,22.23 29.72,21.59 29.72,19.81 v32,17.53 | U2.8 24.77,20.95 v24.77,22.23 | v63.5,17.27 63.5,20.07 64.9,21.46 | 64.9,21.46 67.44,24 | 64.9,21.46 v63.5,22.86 v60.96,22.86
  Bottom 0.203: 33.27,16.13 33.27,16.26
  Bottom 0.254: v74.42,37.72 71.63,37.72 71.63,38.1 | v38.1,37.47 v38.1,33.66
  Bottom 0.508: v24.77,22.23 v18.41,22.23 | v5.71,31.75 5.71,26.67 v3.17,24.13 | v49.53,38.1 49.53,39.88 50.04,40.39 69.6,40.39 71.63,38.35 71.63,38.1 71.63,33.27 69.34,30.99 69.34,27.43 71.98,24.79 v71.98,22.38 | v26.54,34.16 25.4,33.02 v22.86,33.02 | v63.5,17.27 62.48,16.26 v37.85,16.26 33.27,16.26 v32,17.53
VIN
  Top 0.635: D8.A 63.75,43.26 63.75,45.47 J1.20
XI  (via drill 0.5)
  Top 0.254: U1.28 35.04,33.77 v35.56,34.29 | v27.81,38.35 X1.1
  Bottom 0.254: v35.56,34.29 29.84,34.29 27.81,36.32 v27.81,38.35
XO  (via drill 0.5)
  Top 0.254: U1.29 35.1,32.97 v35.56,32.51 | v27.81,28.7 X1.2
  Bottom 0.254: v35.56,32.51 29.84,32.51 27.81,30.48 v27.81,28.7

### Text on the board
Bottom: 10/12 | KWA
tPlace: P01 | P03 | P05 | P07 | P09 | P11 | P13 | P15 | P17 | P19 | P21 | P23 | P25 | P27 | USB | XIO | RTS | CTS | REG | VIN | TV | P00 | P02 | P04 | P06 | P08 | P10 | P12 | P14 | P16 | P18 | P20 | P22 | P24 | P26 | SDA | SCL | TXO | RXI | RES | GND | USER | CD | DO | DI | CK | CS | RX | LED | uSD | TX | BTN | AUX | 6MHz | SDA | PAN | PWR | SCK | TLT | 2.8 | GND | GND | 3.0 | 3.0 | CMUcam4 | CAMERA | www.cmucam.org | 9V MAX | 64KB | + | GND | N/C | N/C | N/C | Y00 | GND | XCK | GND | GND | SCL | SDA | PWD | Y08 | Y06 | Y04 | Y02 | PAN | TLT | - | N/C | N/C | N/C | N/C | Y01 | PWR | PWR | PCK | VSY | HRF | N/C | RST | Y09 | Y07 | Y05 | Y03 | SIG | SIG | SERVO PWR | PWR | GND | PWR | PWR | TXO | RXI | DTR | GND | DTR | TXO | RXI | VCC | CTS | GND | GND | GND | RES
bPlace: P01 | P03 | P05 | P07 | P09 | P11 | P13 | P15 | P17 | P19 | P21 | P23 | P25 | P27 | USB | XIO | RTS | CTS | REG | VIN | P00 | P02 | P04 | P06 | P08 | P10 | P12 | P14 | P16 | P18 | P20 | P22 | P24 | P26 | SDA | SCL | TXO | RXI | RES | GND | CD | DO | DI | CK | CS | RX | LED | TX | BTN | AUX | SDA | PAN | PWR | SCK | TLT | 2.8 | GND | GND | 3.0 | 3.0 | REVA | + | GND | N/C | N/C | N/C | Y00 | GND | XCK | GND | GND | SCL | SDA | PWD | Y08 | Y06 | Y04 | Y02 | PAN | TLT | - | N/C | N/C | N/C | N/C | Y01 | PWR | PWR | PCK | VSY | HRF | N/C | RST | Y09 | Y07 | Y05 | Y03 | SIG | SIG | TXO | RXI | DTR | GND | DTR | TXO | RXI | VCC | CTS | GND | PWR | GND | PWR | PWR | GND | GND
tDocu: Released under the Creative Commons Attribution Share-Alike 3.0 License | http://creativecommons.org/licenses/by-sa/3.0 | Special thanks to SparkFun Electronics for their Eagle Library

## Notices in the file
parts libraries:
SparkFun-Connectors: Licensing: CC v3.0 Share-Alike You are welcome to use this library for commercial purposes.
